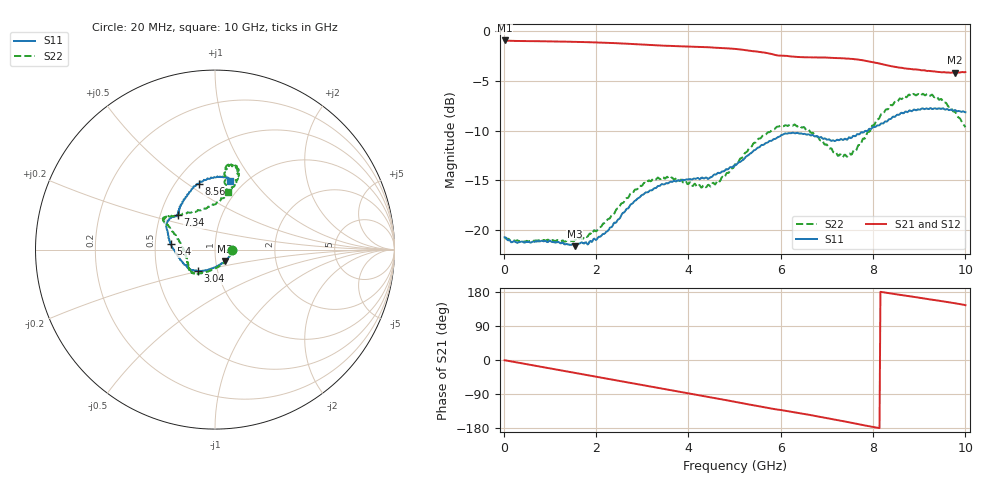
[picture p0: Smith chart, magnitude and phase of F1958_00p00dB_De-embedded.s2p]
! Integrated Device Technology
! Corporate Headquarters
! 6024 Silver Creek Valley Road
! San Jose, CA 95138  USA
! Phone:  1-408-284-8200
! Toll Free:  1-800-223-1366
! Webpage:  http://www.idt.com/
! Timing and RF Division
! 515 Groton Road, Suite 102
! Westford, MA 01886-6024
! Device:  F1958
! Description: 7-bit 0.25 dB Digital Step Attenuator
! Frequency:  0.001 -  6.000 GHz
! Package:  4x4 mm Thin QFN Plastic Package: 24 pin
! Ports:  2 RF, 12 DC
!  Pin  1  = D0
!  Pin  2  = VDD
!  Pin  3  = VMODE
!  Pin  4  = GND
!  Pin  5  = RF1  =  Port 1
!  Pin  6  = GND
!  Pin  7  = GND
!  Pin  8  = GND
!  Pin  9  = GND
!  Pin 10  = GND
!  Pin 11  = GND
!  Pin 12  = GND
!  Pin 13  = GND
!  Pin 14  = RF2  =  Port 2
!  Pin 15  = GND
!  Pin 16  = LE
!  Pin 17  = CLK
!  Pin 18  = DATA
!  Pin 19  = D6
!  Pin 20  = D5
!  Pin 21  = D4
!  Pin 22  = D3
!  Pin 23  = D2
!  Pin 24  = D1
! State:  0
! Atten State:  0.00 dB
! Voltage:  +3.30 Volts
! Current:  0.257 mA
! Data:  The device was measured on a F1958 evaluation board which has
!  individual transmission lines to the RF pins.  Data was collected
!  using a calibrated network analyzer.  The evaluation board was
!  de-embedded using Automatic Fixture Removal (AFR).
!  The reference plane is the edge of the package pin.
! Misc:
!  Action Tracker AT0419
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# GHz S dB R 50
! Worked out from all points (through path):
!   500 points, 20 MHz to 10 GHz, reference 50 ohm
!   highest |S21| = -0.97 dB at 20 MHz (marker M1); lowest = -4.2 dB at 9.78 GHz (marker M2)
!   group delay of S21, straight-line fit = 60.4 ps
!   lowest |S11| = -21.6 dB at 1.54 GHz (marker M3), VSWR 1.18, Z = 55.1 - j7.12 ohm
!   |S11| at or under -10 dB: start of sweep to 7.887 GHz
!   |S22| runs from -21.2 to -6.3 dB; largest |S21 - S12| = 0.0025
!   S11 on the Smith chart (normalised r, x): 20 MHz: 1.20, -0.01; 3.04 GHz: 0.80, -0.20; 5.4 GHz: 0.60, +0.04; 7.34 GHz: 0.62, +0.26; 8.56 GHz: 0.65, +0.55; 10 GHz: 0.86, +0.77
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0.02  -20.70 -1.8  -0.97 -0.6  -0.97 -0.6  -20.70 -2.0
0.3  -21.25 -6.6  -1.02 -6.7  -1.03 -6.7  -20.99 -8.4
0.8  -21.09 -18.1  -1.05 -17.6  -1.05 -17.5  -21.04 -21.3
1.54  -21.59 -50.4  -1.12 -33.9  -1.11 -33.8  -20.97 -57.3
1.7  -21.23 -59.3  -1.13 -37.3  -1.13 -37.3  -20.89 -66.2
2.22  -20.15 -90.5  -1.21 -48.8  -1.20 -48.7  -19.13 -95.2
3.04  -16.36 -128.8  -1.40 -67.0  -1.39 -67.0  -15.25 -128.6
3.36  -15.56 -135.5  -1.48 -73.9  -1.48 -74.0  -14.77 -135.0
4.44  -14.83 -151.3  -1.65 -97.5  -1.67 -97.5  -15.44 -169.1
5.02  -13.46 -171.6  -1.82 -110.6  -1.84 -110.6  -13.35 164.3
5.4  -12.06 172.8  -2.05 -119.3  -2.06 -119.3  -11.36 155.2
5.98  -10.59 155.9  -2.49 -131.6  -2.51 -131.5  -9.55 149.9
6.34  -10.24 147.1  -2.62 -139.0  -2.63 -138.9  -9.56 148.5
6.68  -10.45 142.0  -2.67 -146.0  -2.69 -145.9  -10.22 142.2
7.34  -10.94 136.8  -2.76 -161.2  -2.77 -161.1  -12.67 109.6
7.6  -10.57 133.0  -2.86 -167.2  -2.85 -167.2  -11.96 92.7
8.02  -9.63 121.8  -3.17 -177.2  -3.18 -177.2  -9.48 76.1
8.34  -8.90 111.6  -3.49 176.4  -3.50 176.3  -7.77 72.1
8.56  -8.44 104.0  -3.69 172.3  -3.70 172.4  -6.88 72.8
9.26  -7.79 84.2  -4.05 159.4  -4.06 159.4  -6.43 80.5
9.78  -7.95 78.1  -4.21 149.7  -4.22 149.7  -8.15 81.6
10  -8.16 78.1  -4.14 144.7  -4.17 144.9  -9.67 77.7
